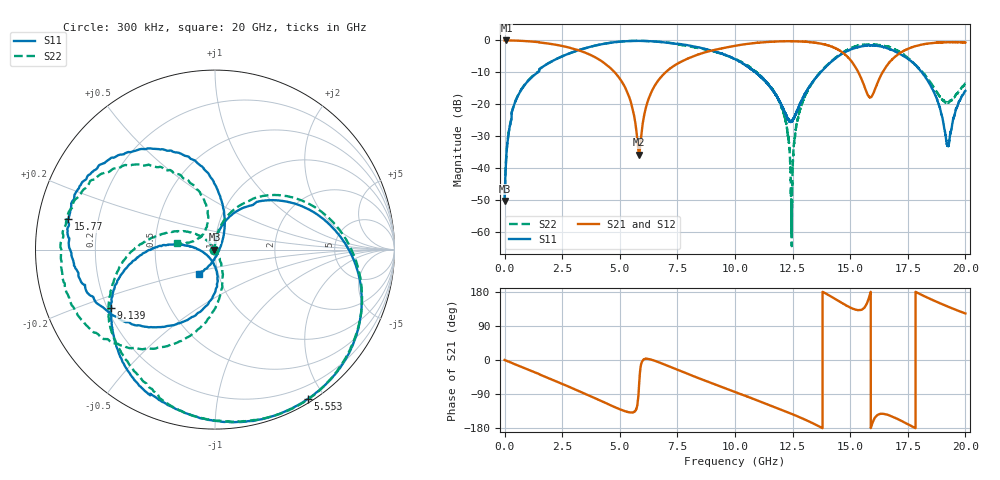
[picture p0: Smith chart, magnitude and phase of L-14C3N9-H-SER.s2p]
!{L-14C3N9}
!Johanson Technology Inc.
!www.johansontechnology.com
!Test Board Conditions:
!Substrate Type  RO4350B
!Substrate Thickness  20 mil
!Substrate Dk  3.66
!TL Type: GCPW
!TL Trace Width  36 mil
!TL Gap  12 mil
!Electrode orientation  Horizontal
!DUT TOPOLOGY	SERIES
!Mounting Pad LxW  26x36 mil
! Created Sun Jun 20 12:56:58 2021
# hz S ma R 50
! 2 Port Network Data from SP1.SP block
! freq  magS11  angS11  magS21  angS21  magS12  angS12  magS22  angS22
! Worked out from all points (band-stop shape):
!   20001 points, 300 kHz to 20 GHz, reference 50 ohm
!   highest |S21| = -0.01 dB at 82.3 MHz (marker M1); lowest = -35.8 dB at 5.838 GHz (marker M2)
!   |S21| within 3 dB of the highest: start of sweep to 3.176 GHz; 9.099 GHz to 14.51 GHz (5.408 GHz wide, 45.8 % of centre)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
!   lowest |S11| = -50.3 dB at 1.3 MHz (marker M3), VSWR 1.01, Z = 49.7 + j0.0161 ohm
!   |S11| at or under -10 dB: start of sweep to 1.445 GHz; 10.9 GHz to 13.71 GHz (2.816 GHz wide, 22.9 % of centre); 18.11 GHz to end of sweep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
!   |S22| runs from -64.5 to -0.1 dB; largest |S21 - S12| = 0.013
!   S11 on the Smith chart (normalised r, x): 300 kHz: 0.99, -0.00; 5.553 GHz: 0.04, -1.80; 9.139 GHz: 0.22, -0.25; 15.77 GHz: 0.09, +0.10; 20 GHz: 0.81, -0.22
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300000  0.003118 -178.2  0.9976 -0.0  0.9959 0.0  0.003208 -172.8
1300000  0.00304 176.9  0.997 -0.1  0.9969 -0.0  0.003132 172.6
8.23e7  0.01699 94.4  0.9983 -2.1  0.9971 -2.1  0.01729 95.2
3.633e8  0.08606 80.2  0.9958 -9.2  0.9953 -9.2  0.08726 81.7
7.803e8  0.1802 68.6  0.9817 -19.4  0.9813 -19.5  0.1825 71.5
3.3343e9  0.7262 2.6  0.6762 -85.0  0.6769 -85.0  0.7255 5.6
5.5533e9  0.9791 -58.2  0.08616 -138.6  0.08625 -138.6  0.9836 -58.9
5.8383e9  0.9827 -66.6  0.01618 -64.5  0.01648 -64.8  0.9846 -66.9
6.6673e9  0.9525 -91.0  0.2351 -5.6  0.2353 -5.2  0.9513 -90.2
9.1393e9  0.6641 -150.6  0.7136 -64.5  0.7158 -64.9  0.6647 -153.0
1.00003e10  0.5102 -167.7  0.8217 -84.5  0.8251 -84.5  0.5125 -173.1
1.18823e10  0.1199 174.6  0.9627 -128.2  0.9634 -128.2  0.1184 138.4
1.22393e10  0.06551 -165.2  0.9699 -136.8  0.9702 -136.9  0.04588 130.6
1.24503e10  0.05436 -129.6  0.9696 -142.0  0.9716 -142.1  0.001998 60.6
1.27403e10  0.08568 -93.0  0.9649 -149.4  0.9668 -149.4  0.06075 -64.4
1.33343e10  0.2151 -88.2  0.9345 -165.7  0.9373 -165.7  0.2116 -79.0
1.46573e10  0.6238 -138.4  0.6512 150.0  0.6538 149.8  0.6356 -120.5
1.57653e10  0.8348 168.2  0.1394 155.4  0.1399 154.5  0.8617 -167.7
1.66673e10  0.7374 134.0  0.4383 -145.5  0.4337 -144.3  0.7957 152.0
1.83283e10  0.2461 79.6  0.8887 165.3  0.8901 165.4  0.2618 101.5
1.92283e10  0.02287 -20.9  0.9371 141.2  0.9375 141.4  0.1073 138.4
2e10  0.162 -123.4  0.9286 122.8  0.9231 122.5  0.2119 170.7
